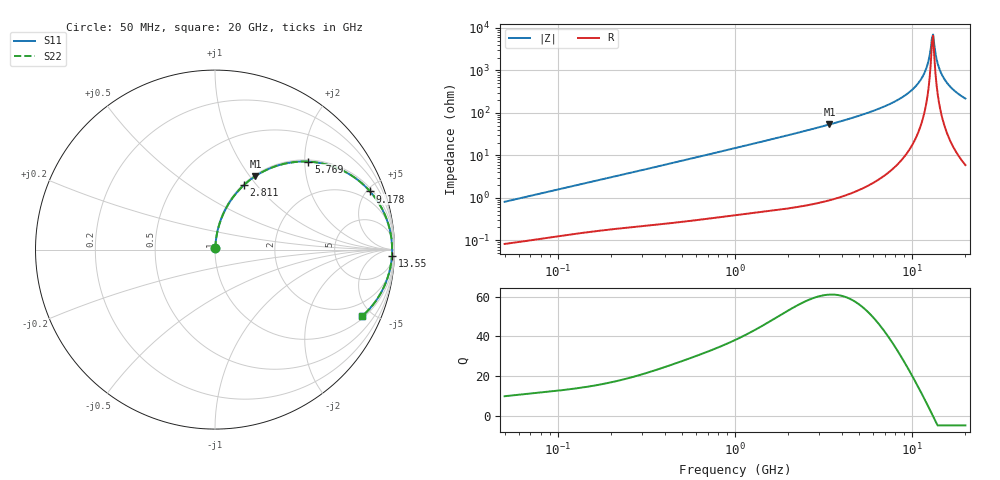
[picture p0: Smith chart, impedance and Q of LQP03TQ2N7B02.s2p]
!Murata Part Number: LQP03TQ2N7B02
!These Parameters are Measured in Series Mode Connection
!  o--[Z]--o
!Port1  Port2
!  o-------o
!Freq. Start=50[MHz] Stop=20[GHz], 401[Steps]
# Hz S RI R 50
!Freq.(Hz) S11(Real) S11(Imag) S21(Real) S21(Imag) S12(Real) S12(Imag) S22(Real) S22(Imag)
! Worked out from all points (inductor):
!   401 points, 50 MHz to 20 GHz, reference 50 ohm
!   read as one part in series: L = 2.52 nH near 51.52 MHz
!   highest Q = 61.2 at 3.415 GHz (marker M1), where L = 2.48 nH
!   self-resonance near 12.95 GHz
!   S11 on the Smith chart (normalised r, x): 50 MHz: 1.00, +0.02; 2.811 GHz: 1.01, +0.86; 5.769 GHz: 1.04, +2.08; 9.178 GHz: 1.20, +5.24; 13.55 GHz: 18, -48; 20 GHz: 1.12, -4.34
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5e7  0.000881 0.00799  0.9991 -0.00799  0.9991 -0.00799  0.000881 0.00799
1.364002e8  0.00192 0.0209  0.9981 -0.0209  0.9981 -0.0209  0.00192 0.0209
3.721004e8  0.0054 0.0551  0.9946 -0.0551  0.9946 -0.0551  0.0054 0.0551
1e9  0.0249 0.1434  0.9751 -0.1434  0.9751 -0.1434  0.0249 0.1434
2.728004e9  0.1512 0.3499  0.8488 -0.3499  0.8488 -0.3499  0.1512 0.3499
2.810964e9  0.1596 0.3579  0.8404 -0.3579  0.8404 -0.3579  0.1596 0.3579
3.415248e9  0.2251 0.4095  0.7749 -0.4095  0.7749 -0.4095  0.2251 0.4095
5.769027e9  0.5196 0.49  0.4804 -0.49  0.4804 -0.49  0.5196 0.49
7.442007e9  0.7137 0.4394  0.2863 -0.4394  0.2863 -0.4394  0.7137 0.4394
9.178299e9  0.8639 0.3243  0.1361 -0.3243  0.1361 -0.3243  0.8639 0.3243
1.050288e10  0.9368 0.2153  0.0632 -0.2153  0.0632 -0.2153  0.9368 0.2153
1.149051e10  0.9689 0.1309  0.0311 -0.1309  0.0311 -0.1309  0.9689 0.1309
1.220001e10  0.9816 0.0713  0.0184 -0.0713  0.0184 -0.0713  0.9816 0.0713
1.276073e10  0.9862 0.0256  0.0138 -0.0256  0.0138 -0.0256  0.9862 0.0256
1.295331e10  0.9868 0.0103  0.0132 -0.0103  0.0132 -0.0103  0.9868 0.0103
1.314879e10  0.9869 -0.0051  0.0131 0.0051  0.0131 0.0051  0.9869 -0.0051
1.334722e10  0.9866 -0.0204  0.0134 0.0204  0.0134 0.0204  0.9866 -0.0204
1.354865e10  0.9857 -0.0358  0.0143 0.0358  0.0143 0.0358  0.9857 -0.0358
1.417136e10  0.9804 -0.0814  0.0196 0.0814  0.0196 0.0814  0.9804 -0.0814
1.527346e10  0.9622 -0.1553  0.0378 0.1553  0.0378 0.1553  0.9622 -0.1553
1.721783e10  0.9114 -0.2633  0.0886 0.2633  0.0886 0.2633  0.9114 -0.2633
2e10  0.8187 -0.372  0.1813 0.372  0.1813 0.372  0.8187 -0.372
